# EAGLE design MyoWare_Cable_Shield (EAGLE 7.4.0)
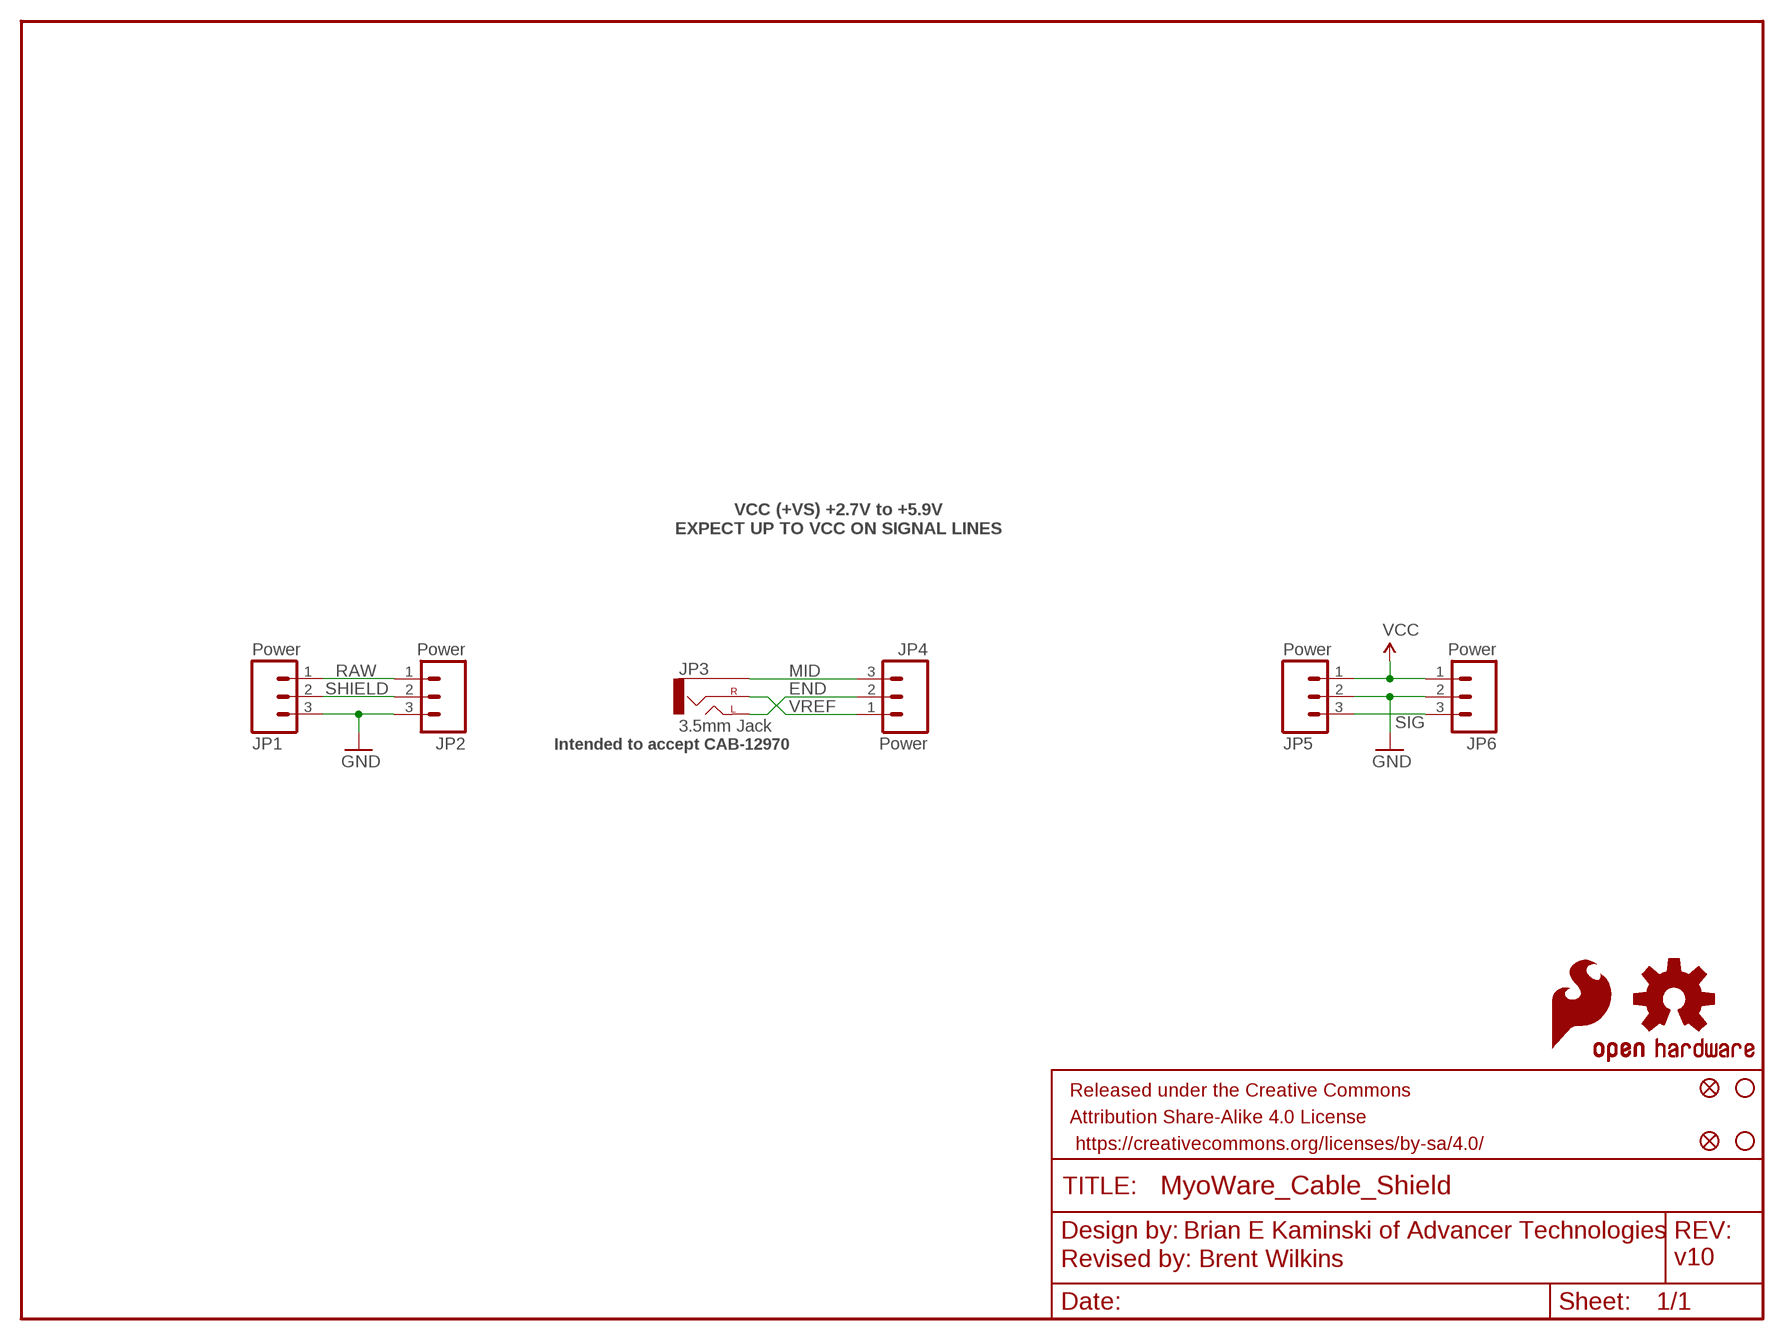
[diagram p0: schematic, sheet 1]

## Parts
FID1  FIDUCIAL1X2  [FIDUCIAL-1X2]
FID2  FIDUCIAL1X2  [FIDUCIAL-1X2]
FRAME1  FRAME-LETTER  [CREATIVE_COMMONS]
JP1  Power  M031X03_NO_SILK  [1X03_NO_SILK]
JP2  Power  M031X03_NO_SILK  [1X03_NO_SILK]
JP3  3.5mm Jack  AUDIO-JACKSMD2  [AUDIO-JACK-3.5MM-SMD]
JP4  Power  M031X03_NO_SILK  [1X03_NO_SILK]
JP5  Power  M031X03_NO_SILK  [1X03_NO_SILK]
JP6  Power  M031X03_NO_SILK  [1X03_NO_SILK]
LOGO1  SFE_LOGO_FLAME.2_INCH  [SFE_LOGO_FLAME_.2]
LOGO2  OSHW-LOGOM  [OSHW-LOGO-M]
STANDOFF1  STAND-OFF  [STAND-OFF]
STANDOFF2  STAND-OFF  [STAND-OFF]

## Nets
END: JP3.TIP(LEFT) JP4.2
GND: JP1.3 JP2.3 JP5.2 JP6.2
MID: JP3.SLEEVE JP4.3
RAW: JP1.1 JP2.1
SHIELD: JP1.2 JP2.2
SIG: JP5.3 JP6.3
VCC: JP5.1 JP6.1
VREF: JP3.RING(RIGHT) JP4.1

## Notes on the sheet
- VCC (+VS) +2.7V to +5.9V
  EXPECT UP TO VCC ON SIGNAL LINES
- Intended to accept CAB-12970
- Brian E Kaminski of Advancer Technologies
- Revised by: Brent Wilkins | v10

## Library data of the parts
FID1 FID2 = SparkFun-Aesthetics:FIDUCIAL: Fiducial Alignment Points
FRAME1 = SparkFun-Aesthetics:FRAME-LETTER: Schematic Frame
JP1 JP2 JP4-JP6 = SparkFun-Connectors:M03: Header 3 Standard 3-pin 0.1" header. Use with straight break away headers (SKU : PRT-00116), right angle break away headers (PRT-00553), swiss pins (PRT-00743), machine pins (PRT-00117), and female headers (PRT-00115). Molex polarized connector foot print use with SKU : PRT-08232 with associated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
JP3 = SparkFun-Connectors:AUDIO-JACK: 3.5mm Audio Jack Simple 3.5mm common PCB mount audio jack. Variant PTH is our storefront SKU PRT-08032; PROD_ID: CONN-10353
LOGO1 = SparkFun-Aesthetics:SFE_LOGO_FLAME: SFE Logo, flame only
LOGO2 = SparkFun-Aesthetics:OSHW-LOGO: Open Source Hardware Logo
STANDOFF1 STANDOFF2 = SparkFun-Electromechanical:STAND-OFF: #4 Stand Off

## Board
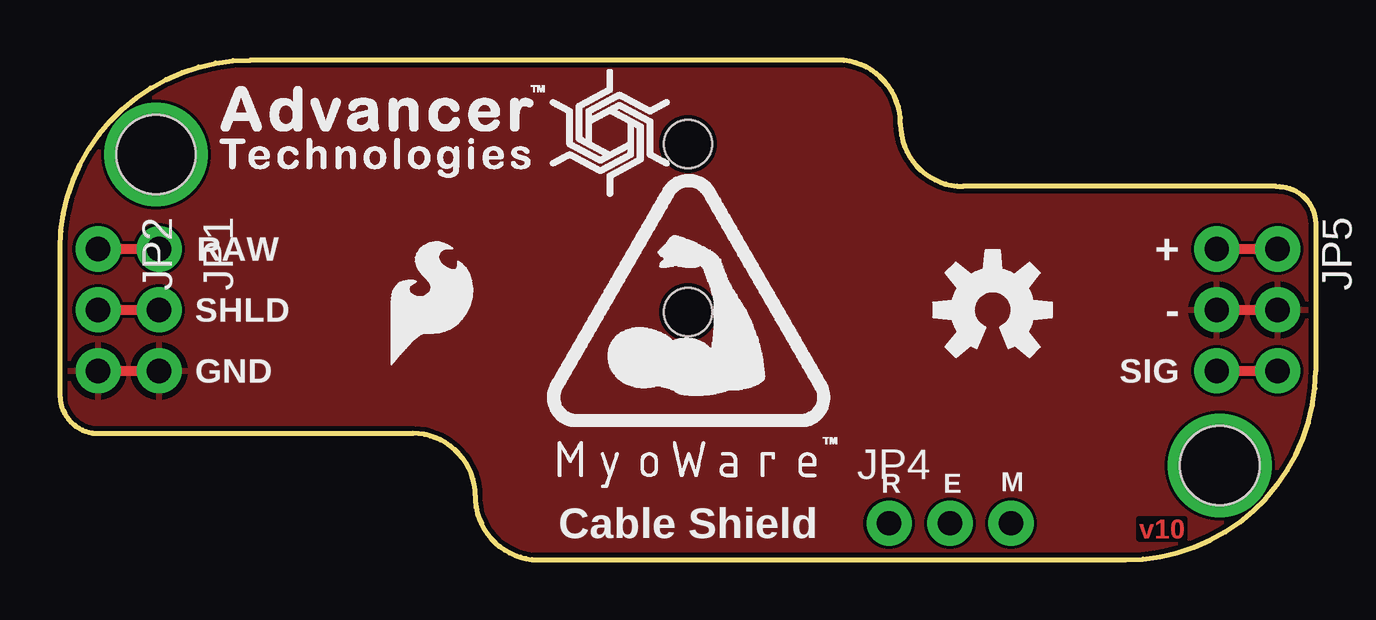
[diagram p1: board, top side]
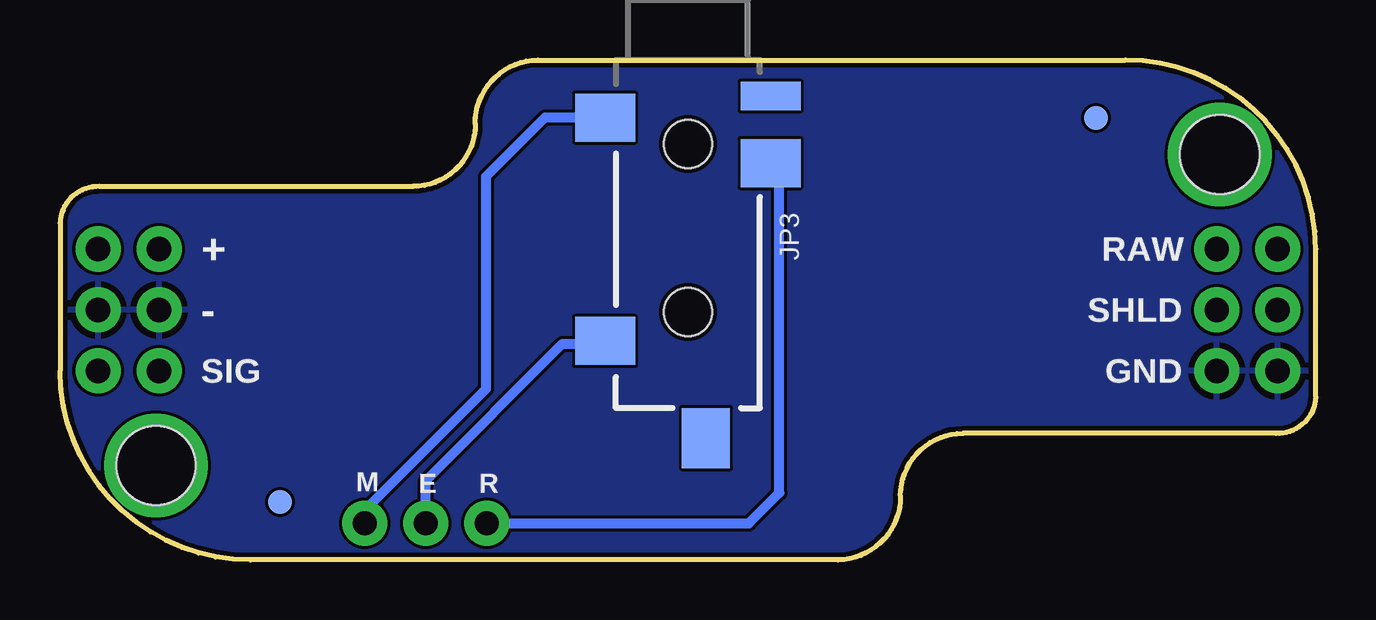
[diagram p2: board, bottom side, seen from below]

Size 52.32 x 20.83 mm. Coordinates in mm from the lower left corner, seen from the top.
Outline: 19.91,0 44.39,0 arc90 52.32,7.87 52.32,14.03 arc90 50.67,15.56 37.62,15.56 arc-90 35.02,18.16 arc90 32.42,20.83 7.94,20.83 arc90 0,12.95 0,6.79 arc90 1.65,5.27 14.7,5.27 arc-90 17.3,2.67 arc90 19.91,0
Copper layers (1*16): Top 0.035mm / dielectric 1.5mm / Bottom 0.035mm
Design rules "Gold_Phoenix_Standard_Spec_2_layer": minimum track width 5mil, minimum drill 6mil, track to track 5mil, track to pad 5mil, pad to pad 5mil, via to via 5mil, smd to smd 5mil, copper to edge 8mil, drill to drill 8mil, minimum pad ring 5mil, minimum via ring 5mil, stop-mask expansion 4mil, vias tented up to drill 20mil, thermal gap 10mil

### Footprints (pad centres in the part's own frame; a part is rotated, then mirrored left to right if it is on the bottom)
FIDUCIAL-1X2 = smd 1 x 1: 1 0,0
1X03_NO_SILK = drill 1.016 pad 1.88: 1 0,0; 2 2.54,0; 3 5.08,0
AUDIO-JACK-3.5MM-SMD = smd 2 x 2.5: RING 4.3,3.45; SLEEVE 2.4,-3.45; TIP 11.7,-3.45 | smd 1.2 x 2.5: RSH 1.5,3.45 | smd 2.5 x 2: TSH 15.75,0.75 | hole 2: 3.5,0; 10.5,0
STAND-OFF = hole 3.302: 0,0

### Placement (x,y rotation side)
FID1  43.16,2.41 0 bottom
FID2  9.16,18.41 0 bottom
FRAME1  not placed on the board
JP1  4.13,12.95 270 top
JP2  1.59,12.95 270 top
JP3  26.16,20.83 270 bottom
JP4  34.54,1.52 0 top
JP5  50.74,12.95 270 top
JP6  48.2,12.95 270 top
LOGO  [MYOWARE_LOGO]  26.16,9.53 0 top
LOGO1  13.46,7.87 0 top
LOGO2  38.86,10.41 0 top
SPIRAL  [SPIRAL_LOGO_60%]  22.95,17.79 0 top
STANDOFF1  4,16.89 0 top
STANDOFF2  48.32,3.94 0 top
U$6  [ADVANCER_LOGO]  13.07,17.64 0 top

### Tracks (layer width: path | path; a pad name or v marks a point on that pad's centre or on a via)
END
  Bottom 0.406: JP3.TIP 29.61,9 31.39,9 37.08,3.3 JP4.2
GND
  Top 0.406: JP6.2 JP5.2 | JP2.3 JP1.3
  pour Top: 0.13,0.06 52.2,0.06 52.2,20.76 0.13,20.76
  pour Bottom: 0.13,0.06 52.2,0.06 52.2,20.76 0.13,20.76
MID
  Bottom 0.406: JP3.SLEEVE 32.12,18.43 34.58,15.97 34.58,7.11 39.62,2.06 JP4.3
N$1  (via drill 3.3)
  other vias: 4,16.89
N$2  (via drill 3.3)
  other vias: 48.32,3.94
RAW
  Top 0.406: JP2.1 JP1.1
SHIELD
  Top 0.406: JP2.2 JP1.2
SIG
  Top 0.406: JP6.3 JP5.3
VCC
  Top 0.406: JP6.1 JP5.1
VREF
  Bottom 0.406: JP4.1 23.62,1.52 22.35,2.79 22.35,16.39 22.49,16.53 JP3.RING

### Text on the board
Top: v10
tPlace: RAW | + | SHLD | - | GND | SIG | R | E | M | Cable Shield
bPlace: RAW | + | SHLD | - | GND | SIG | R | E | M
Measures: All units in inches
tDocu: Brian E Kaminski of Advancer Technologies | Revised by: Brent Wilkins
